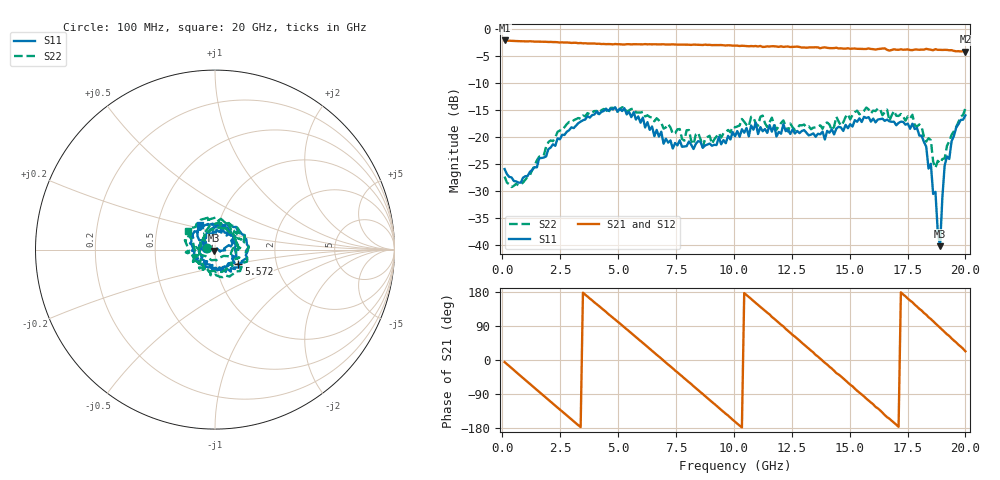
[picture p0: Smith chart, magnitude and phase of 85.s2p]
!Agilent Technologies,N5230C,MY49001569,A.09.33.09
!Agilent N5230C: A.09.33.09
!Date: Tuesday, July 21, 2015 13:22:11
!Correction: S11(Full 2 Port(1,2))
!S21(Full 2 Port(1,2))
!S12(Full 2 Port(1,2))
!S22(Full 2 Port(1,2))
!S2P File: Measurements: S11, S21, S12, S22:
# Hz S  dB  R 50
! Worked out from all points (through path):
!   201 points, 100 MHz to 20 GHz, reference 50 ohm
!   highest |S21| = -2.06 dB at 100 MHz (marker M1); lowest = -4.1 dB at 20 GHz (marker M2)
!   group delay of S21, straight-line fit = 146 ps
!   lowest |S11| = -40.3 dB at 18.91 GHz (marker M3), VSWR 1.02, Z = 49.2 - j0.561 ohm
!   |S11| at or under -10 dB: start of sweep to end of sweep
!   |S22| runs from -29.3 to -14.5 dB; largest |S21 - S12| = 0.028
!   S11 on the Smith chart (normalised r, x): 100 MHz: 0.91, +0.02; 5.572 GHz: 1.28, -0.21; 20 GHz: 0.82, +0.22
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1e8  -25.95 170.4  -2.06 -5.5  -2.01 -5.7  -27.33 170.6
7.965e8  -28.47 162.6  -2.21 -42.3  -2.19 -42.2  -28.76 155.1
1.692e9  -23.89 150.1  -2.29 -89.3  -2.30 -89.2  -23.57 147.7
2.687e9  -19.61 112.5  -2.45 -141.2  -2.43 -141.1  -18.15 109.0
3.483e9  -16.89 76.9  -2.60 177.6  -2.59 177.8  -16.01 73.0
4.5775e9  -15.15 18.1  -2.73 121.5  -2.73 121.9  -15.61 15.3
5.5725e9  -16.30 -31.6  -2.80 70.8  -2.75 71.2  -14.80 -39.0
6.7665e9  -19.90 -88.8  -2.80 9.0  -2.77 9.2  -16.91 -100.8
8.458e9  -20.77 165.6  -2.86 -79.5  -2.87 -78.9  -19.21 177.6
1.005e10  -19.86 76.2  -3.03 -162.6  -3.01 -162.0  -18.19 82.4
1.09455e10  -17.35 33.0  -3.09 150.7  -3.14 151.7  -17.46 41.1
1.1841e10  -19.90 -19.1  -3.19 103.6  -3.21 104.7  -18.65 -3.0
1.3433e10  -19.32 -97.6  -3.35 19.8  -3.30 20.2  -18.25 -99.7
1.4229e10  -18.53 -147.2  -3.49 -22.4  -3.41 -21.9  -18.71 -141.1
1.5224e10  -16.86 166.3  -3.55 -75.5  -3.70 -74.4  -15.38 165.2
1.67165e10  -17.08 96.4  -3.94 -154.9  -3.85 -154.2  -16.98 76.7
1.77115e10  -17.52 40.0  -3.86 152.5  -3.86 152.8  -15.86 37.6
1.83085e10  -21.78 17.7  -3.63 119.5  -3.78 120.7  -20.85 -10.8
1.87065e10  -30.18 -21.6  -3.68 96.5  -3.78 97.4  -25.72 -60.5
1.89055e10  -40.26 -144.0  -3.80 85.5  -3.85 86.3  -24.84 -90.4
1.91045e10  -25.29 164.8  -3.80 73.6  -3.92 74.7  -23.98 -144.7
2e10  -15.98 122.3  -4.13 23.1  -4.22 25.6  -14.66 144.9
